PROGRAM MAIN_CM
VAR CONSTANT
	cInitIntRMS 	: ST_CM_IntegratedRMS_InitPars   := (	nFFT_Length := cFFTLength, 
															nWindowLength := cWindowLength,
															fSampleRate := cFSample,
		 													fLowerFrequencyLimit := cfLowerFrequencyLimit,
															fUpperFrequencyLimit := cfUpperFrequencyLimit,
															nOrder := cOrderRMS,
															nChannels := cChannels,                        
															eWindowType := E_CM_WindowType.eCM_HannWindow, 
															bTransformToDecibel:= FALSE);								
END_VAR

VAR	
	fbRMS				: FB_CMA_IntegratedRMS  	  :=(	stInitPars := cInitIntRMS, 
															nOwnID := eID_IntRMS, 
															aDestIDs := [eID_Sink] );

	fbErrHist			: FB_HRErrHist; // error monitoring

END_VAR

// Call RMS
fbRMS.Call();
IF fbRMS.bError THEN
	fbErrHist.AddError(bErr:=TRUE, hrErrCode:=fbRMS.hrErrorCode, sErrSource:='MAIN_CM.fbRMS'); // error monitoring
	// ToDo: if error
END_IF

END_PROGRAM
